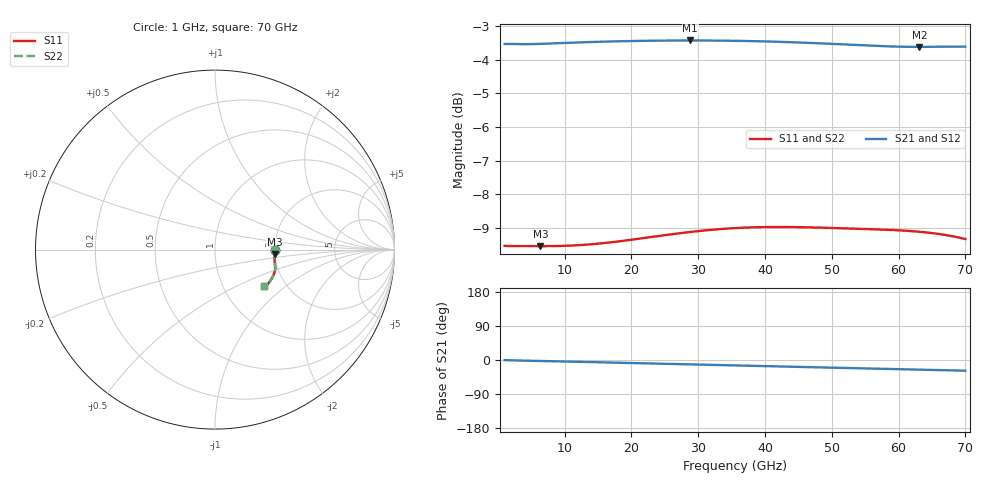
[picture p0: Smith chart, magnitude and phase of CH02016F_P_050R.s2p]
# GHz S RI R 50
! S-Parameters data
! Freq  reS11  imS11  reS21  imS21  reS12  imS12  reS22  imS22
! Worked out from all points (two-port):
!   401 points, 1 GHz to 70 GHz, reference 50 ohm
!   highest |S21| = -3.42 dB at 28.77 GHz (marker M1); lowest = -3.6 dB at 63.1 GHz (marker M2)
!   |S21| within 3 dB of the highest: start of sweep to end of sweep
!   lowest |S11| = -9.6 dB at 6.348 GHz (marker M3), VSWR 2.00, Z = 99.5 - j5.53 ohm
!   |S11| at or under -10 dB: nowhere
!   |S22| runs from -9.5 to -9.0 dB; largest |S21 - S12| = 0
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1  0.3334 -0.00398  0.6666 -0.00453  0.6666 -0.00453  0.3334 -0.00401
3.07  0.3328 -0.0123  0.6659 -0.0154  0.6659 -0.0154  0.3328 -0.0124
6.3475  0.332 -0.0247  0.6661 -0.0292  0.6661 -0.0292  0.3322 -0.0248
9.625  0.3312 -0.0365  0.6673 -0.0438  0.6673 -0.0438  0.3316 -0.0367
12.5575  0.331 -0.0467  0.6679 -0.0576  0.6679 -0.0576  0.3316 -0.0469
17.215  0.3318 -0.0627  0.6676 -0.0803  0.6676 -0.0803  0.3326 -0.0627
20.665  0.3329 -0.0742  0.6665 -0.0971  0.6665 -0.0971  0.3338 -0.0742
24.115  0.3341 -0.0854  0.6646 -0.1137  0.6646 -0.1137  0.335 -0.0853
28.7725  0.3351 -0.0995  0.6608 -0.1357  0.6608 -0.1357  0.3359 -0.0993
32.2225  0.3349 -0.1095  0.6571 -0.1517  0.6571 -0.1517  0.3356 -0.1092
35.5  0.3337 -0.1188  0.6529 -0.1667  0.6529 -0.1667  0.3343 -0.1185
38.26  0.3318 -0.1267  0.6487 -0.1793  0.6487 -0.1793  0.3323 -0.1265
41.02  0.329 -0.1348  0.644 -0.1918  0.644 -0.1918  0.3295 -0.1346
43.9525  0.3252 -0.1437  0.6385 -0.205  0.6385 -0.205  0.3258 -0.1435
47.0575  0.3203 -0.1531  0.632 -0.2186  0.632 -0.2186  0.3211 -0.1531
53.2675  0.3092 -0.1716  0.6177 -0.2443  0.6177 -0.2443  0.3102 -0.1715
58.615  0.299 -0.1859  0.6054 -0.2652  0.6054 -0.2652  0.3001 -0.1857
63.1  0.2897 -0.1962  0.5959 -0.2835  0.5959 -0.2835  0.2907 -0.1958
65.17  0.2849 -0.2  0.5918 -0.2924  0.5918 -0.2924  0.2859 -0.1996
66.895  0.2807 -0.2025  0.5884 -0.2998  0.5884 -0.2998  0.2816 -0.2021
68.965  0.2756 -0.2043  0.5842 -0.3083  0.5842 -0.3083  0.2763 -0.2039
70  0.273 -0.2046  0.5821 -0.3122  0.5821 -0.3122  0.2737 -0.2042
